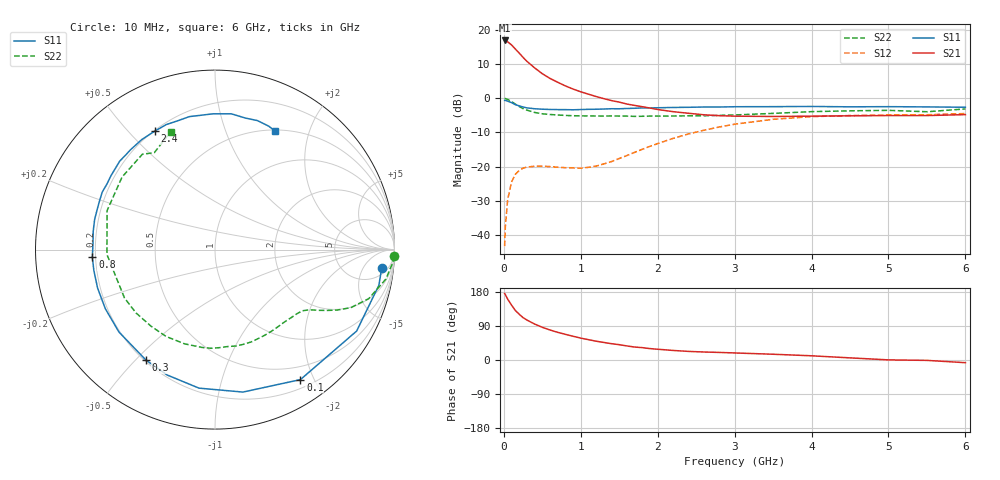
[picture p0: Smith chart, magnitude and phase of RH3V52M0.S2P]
! SIEMENS Small Signal Semiconductors
! BFR106
! Si NPN RF Bipolar Junction Transistor in SOT23
! VCE = 3.5 V  IC = 2 mA
! Common Emitter S-Parameters:  August  1996
# GHz  S  MA  R  50
!  f  S11  S21  S12  S22
! GHz  MAG  ANG  MAG  ANG  MAG  ANG  MAG  ANG
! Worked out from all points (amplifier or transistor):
!   36 points, 10 MHz to 6 GHz, reference 50 ohm
!   highest |S21| = 17.0 dB at 10 MHz (marker M1)
!   |S21| within 3 dB of that: start of sweep to 170.1 MHz
!   unconditionally stable (mu >= 1): 782 MHz to 1.954 GHz; 3.801 GHz to end of sweep
!   at 250 MHz: K = 0.33, MSG = 16.2 dB, |S12| = -20.5 dB
!   at 1.4 GHz: K = 1.27, MAG = 5.8 dB, |S12| = -18.5 dB
!   at 6 GHz: K = 1.02, MAG = -1.1 dB, |S12| = -4.4 dB
!   S11 on the Smith chart (normalised r, x): 10 MHz: 8, -13; 100 MHz: 0.31, -1.81; 300 MHz: 0.21, -0.54; 800 MHz: 0.19, -0.03; 2.4 GHz: 0.20, +0.59; 6 GHz: 0.51, +1.50
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0.01  0.9347 -6.3  7.077 175.3  0.0068 87.5  0.999 -2.1
0.02  0.9344 -12.3  7.035 172.3  0.0134 83.5  0.9935 -4.1
0.05  0.9103 -29.9  6.75 160.5  0.0328 73.2  0.966 -9.8
0.1  0.8667 -56.7  6.088 144.9  0.0594 60.6  0.8991 -17.7
0.15  0.8089 -78.9  5.294 130.6  0.0772 49.0  0.8233 -23.1
0.2  0.777 -96.6  4.617 120.7  0.0879 41.8  0.7604 -26.3
0.25  0.7478 -110.9  3.995 111.8  0.0948 35.6  0.708 -28.6
0.3  0.7259 -122.0  3.497 105.4  0.0984 32.3  0.6727 -30.2
0.4  0.7052 -139.4  2.805 94.9  0.1012 27.3  0.6224 -32.6
0.5  0.6941 -151.7  2.301 86.3  0.1013 25.2  0.5945 -35.0
0.6  0.6883 -161.9  1.964 79.2  0.0999 24.9  0.5806 -37.8
0.8  0.6845 -176.5  1.524 67.7  0.0963 29.1  0.5624 -44.3
1.1  0.6913 165.9  1.153 53.6  0.0975 43.4  0.5531 -55.7
1.6  0.7111 144.6  0.826 37.1  0.1452 65.2  0.5498 -77.7
2.2  0.7364 123.7  0.639 25.2  0.2588 65.9  0.5517 -107.8
2.4  0.7404 117.0  0.605 22.7  0.3008 62.8  0.5554 -119.3
3  0.7546 100.9  0.549 18.6  0.4183 49.7  0.5718 -151.8
3.5  0.7567 90.7  0.543 15.2  0.4936 37.7  0.6027 -177.4
4.5  0.7523 77.1  0.555 5.6  0.5606 16.2  0.657 142.0
5  0.7566 71.8  0.56 0.3  0.571 8.0  0.6678 127.3
5.5  0.7502 66.6  0.56 -1.0  0.5757 4.1  0.6373 122.0
6  0.7412 63.4  0.578 -7.1  0.5998 -3.8  0.7008 110.7
